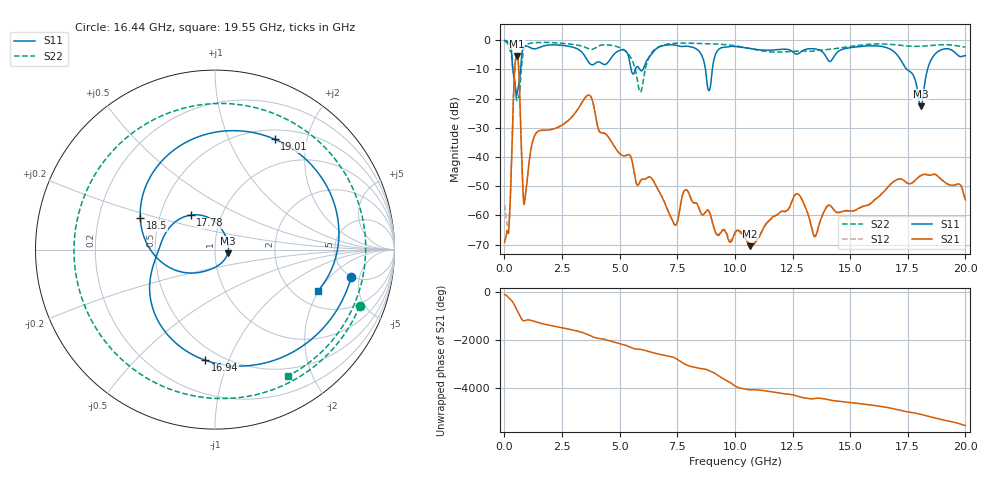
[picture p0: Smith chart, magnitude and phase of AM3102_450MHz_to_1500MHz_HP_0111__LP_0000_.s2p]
!Agilent Technologies,E8364B,MY43040894,A.07.50.67
!Agilent E8364B: A.07.50.67
!Date: Thursday, January 11, 2018 05:50:46
!Correction: S11(Full 2 Port(1,2))
!S21(Full 2 Port(1,2))
!S12(Full 2 Port(1,2))
!S22(Full 2 Port(1,2))
!S2P File: Measurements: S11, S21, S12, S22:
# Hz S  dB  R 50
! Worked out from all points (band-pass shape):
!   1601 points, 10 MHz to 20 GHz, reference 50 ohm
!   highest |S21| = -5.34 dB at 534.7 MHz (marker M1); lowest = -70.6 dB at 10.67 GHz (marker M2)
!   |S21| within 3 dB of the highest: 462.4 MHz to 611.7 MHz (149.3 MHz wide, 27.8 % of centre)
!   lowest |S11| = -22.7 dB at 18.06 GHz (marker M3), VSWR 1.16, Z = 57.5 - j2.46 ohm
!   |S11| at or under -10 dB: 367.7 MHz to 704.8 MHz (337.1 MHz wide, 62.9 % of centre); 8.724 GHz to 9.02 GHz (295.9 MHz wide, 3.34 % of centre); 17.47 GHz to 18.36 GHz (890.6 MHz wide, 4.97 % of centre)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
!   |S22| runs from -20.7 to -0.3 dB; largest |S21 - S12| = 0.0023
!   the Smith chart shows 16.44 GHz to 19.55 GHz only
!   S11 on the Smith chart (normalised r, x): 16.44 GHz: 4.90, -3.77; 16.94 GHz: 0.41, -0.83; 17.78 GHz: 0.71, +0.29; 18.5 GHz: 0.39, +0.17; 19.01 GHz: 0.62, +1.49; 19.55 GHz: 2.62, -1.95
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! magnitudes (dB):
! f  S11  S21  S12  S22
! 10 MHz  -0.1  -69.2  -56.4  -0.3
! 209.9 MHz  -0.8  -62.1  -61.8  -2.8
! 534.7 MHz  -18.9  -5.3  -5.3  -20.7
! 884.6 MHz  -2.0  -54.9  -54.8  -2.1
! 1.359 GHz  -2.9  -32.0  -32.0  -0.8
! 3.346 GHz  -4.0  -21.6  -21.6  -2.0
! 5.895 GHz  -10.2  -48.3  -48.3  -17.8
! 6.682 GHz  -2.4  -51.3  -51.4  -2.3
! 8.881 GHz  -17.3  -58.5  -58.7  -1.2
! 10.01 GHz  -2.1  -66.1  -65.5  -1.9
! 10.67 GHz  -2.9  -70.6  -70.2  -2.8
! 12.68 GHz  -4.8  -52.7  -52.6  -3.7
! 13.34 GHz  -2.9  -64.6  -64.7  -3.8
! 16.44 GHz  -2.2  -52.1  -52.1  -1.3
! 16.68 GHz  -2.8  -50.0  -49.9  -1.4
! 16.94 GHz  -4.2  -48.2  -48.1  -1.5
! 17.78 GHz  -12.6  -48.3  -48.3  -2.1
! 18.06 GHz  -22.7  -46.4  -46.4  -2.1
! 18.5 GHz  -6.9  -46.2  -46.2  -1.8
! 19.01 GHz  -3.1  -48.1  -48.1  -1.5
! 19.55 GHz  -4.2  -49.6  -49.5  -1.8
! 20 GHz  -5.2  -54.6  -54.5  -2.3
